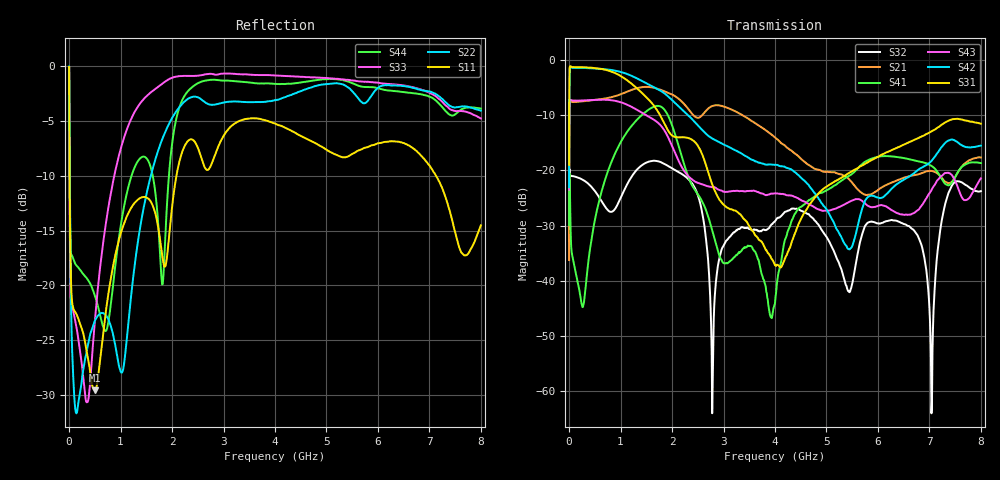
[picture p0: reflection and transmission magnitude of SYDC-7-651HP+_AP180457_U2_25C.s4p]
!Created: 06-20-2018 at 12:38:10
!Mini-Circuits
!S4P DATA File Format
!Type: Directional Coupler
!MODEL: SYDC-7-651HP+
!S/N: Unit 2
!TEST CONDITIONS: Z:50 OHM SYSTEM, INPUT POWER = 0dBm, TEMP:25°C
!REMARK: Full 2 port calibration using Ecal. Port  extension done.
!TESTED ON: NETWORK ANALYZER MODEL E5071C S/N 76113 CAL DUE DATE 05/10/19
# MHZ S DB R 50
!Frequency  S11 dB  S11 DEG  S12 dB  S12 DEG  S13 dB  S13 DEG  S14 dB  S14 DEG
!  S21 dB  S21 DEG  S22 dB  S22 DEG  S23 dB  S23 DEG  S24 dB  S24 DEG
!  S31 dB  S31 DEG  S32 dB  S32 DEG  S33 dB  S33 DEG  S34 dB  S34 DEG
!  S41 dB  S41 DEG  S42 dB  S42 DEG  S43 dB  S43 DEG  S44 dB  S44 DEG
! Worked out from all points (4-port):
!   1501 points, 300 kHz to 8 GHz, reference 50 ohm
!   strongest paths, dB at 300 kHz, 675 kHz, 500 MHz, 4.25 GHz, 8 GHz:
!     S31: -19.0, -12.3, -1.4, -34.7, -11.5
!     S42: -23.1, -16.2, -1.5, -19.6, -15.5
!     S43: -23.5, -16.8, -7.2, -24.5, -21.4
!     S41: -29.9, -23.3, -29.0, -31.0, -18.7
!     S21: -36.2, -28.6, -7.2, -16.0, -17.7
!     S32: -32.9, -26.2, -23.7, -27.3, -23.8
!   lowest |S11| = -29.5 dB at 500 MHz (marker M1), VSWR 1.07, Z = 47.9 - j2.51 ohm
!   |S11| at or under -10 dB: 9.57 MHz to 2.085 GHz (2.076 GHz wide, 198 % of centre); 7.129 GHz to end of sweep
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0.3  -0.08 173.2  -36.30 91.4  -19.00 80.0  -29.86 -101.6
     -36.24 91.6  -0.03 175.8  -32.86 -99.7  -22.95 82.5
     -19.00 80.1  -32.91 -99.9  -0.10 173.0  -23.50 -98.4
     -29.89 -102.1  -23.05 82.1  -23.49 -98.9  -0.10 175.2
120  -22.42 -1.3  -7.59 -1.2  -1.28 -8.8  -38.24 122.4
     -7.59 -1.2  -31.24 18.4  -21.15 165.9  -1.42 -7.2
     -1.29 -8.8  -21.14 165.9  -23.26 166.8  -7.35 163.9
     -38.21 122.2  -1.41 -7.2  -7.35 163.9  -18.02 162.8
500  -29.54 -128.2  -7.23 -14.0  -1.44 -41.5  -29.02 -72.4
     -7.23 -14.0  -23.22 -97.6  -23.73 128.3  -1.54 -36.1
     -1.44 -41.5  -23.75 128.2  -23.25 -72.3  -7.23 110.2
     -29.02 -72.7  -1.53 -36.1  -7.22 110.2  -20.92 136.5
1750  -15.25 -12.5  -5.27 -82.2  -9.65 -159.0  -8.33 26.2
      -5.30 -82.2  -7.44 -58.0  -18.34 56.3  -5.44 -141.5
      -9.71 -158.8  -18.39 56.7  -1.83 -134.6  -11.61 -103.7
      -8.34 26.3  -5.42 -141.5  -11.56 -104.0  -15.72 -128.7
2790  -8.66 -6.8  -8.27 -125.3  -22.69 136.8  -31.14 -159.3
      -8.31 -125.4  -3.54 -120.5  -58.58 86.4  -14.23 146.7
      -22.78 136.9  -58.02 86.9  -0.74 176.0  -23.03 98.9
      -31.17 -159.0  -14.26 146.6  -23.04 98.6  -1.25 -129.1
4070  -5.39 -49.0  -14.61 121.1  -37.07 67.6  -38.14 89.8
      -14.58 120.8  -3.06 -166.5  -28.54 4.4  -19.08 69.4
      -37.24 65.4  -28.59 3.5  -0.88 134.8  -24.17 15.1
      -38.44 87.0  -19.15 69.2  -24.23 15.1  -1.64 167.6
8000  -14.52 -51.0  -17.61 179.1  -11.32 110.6  -18.73 -178.2
      -17.66 178.4  -4.08 41.6  -23.55 -60.5  -15.71 177.6
      -11.53 110.1  -23.75 -59.8  -4.78 -4.2  -21.84 46.6
      -18.67 -178.4  -15.51 178.2  -21.44 47.3  -3.88 30.3
